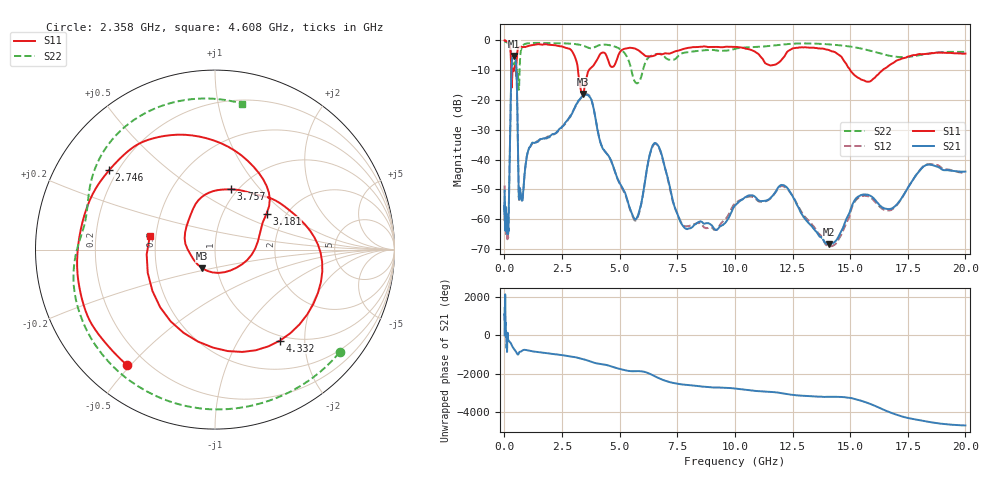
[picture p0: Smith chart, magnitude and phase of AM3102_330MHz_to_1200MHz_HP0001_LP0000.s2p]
! Date/Time: Tue, Sep 11, 2018 5:09 PM
! Network Analyzer: Agilent Technologies E8362B Rev: A.07.50.63
! Sweep from 0.010 to 20.000 GHz, 1601 Points, Sweep Type: LOG
! Power Supply: 4.950 V, 0.000 A
# Hz S DB R 50
!freq MagS11 AngS11 MagS21 AngS21 MagS12 AngS12 MagS22 AngS22
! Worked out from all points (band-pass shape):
!   1601 points, 10 MHz to 20 GHz, reference 50 ohm
!   highest |S21| = -5.20 dB at 399 MHz (marker M1); lowest = -68.4 dB at 14.07 GHz (marker M2)
!   |S21| within 3 dB of the highest: 315.2 MHz to 511 MHz (195.8 MHz wide, 47.4 % of centre)
!   lowest |S11| = -18.0 dB at 3.4 GHz (marker M3), VSWR 1.29, Z = 42.4 - j8.91 ohm
!   |S11| at or under -10 dB: 295.7 MHz to 352.7 MHz (56.97 MHz wide, 17.6 % of centre); 3.192 GHz to 3.661 GHz (469.1 MHz wide, 13.7 % of centre); 15.01 GHz to 16.4 GHz (1.393 GHz wide, 8.87 % of centre)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
!   |S22| runs from -16.6 to -0.2 dB; largest |S21 - S12| = 0.0067
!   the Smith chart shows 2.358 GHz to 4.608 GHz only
!   S11 on the Smith chart (normalised r, x): 2.358 GHz: 0.13, -0.49; 2.746 GHz: 0.17, +0.32; 3.181 GHz: 1.60, +0.73; 3.757 GHz: 0.93, +0.71; 4.332 GHz: 0.92, -1.53; 4.608 GHz: 0.46, +0.08
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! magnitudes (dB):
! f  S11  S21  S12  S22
! 10 MHz  0.0  -50.4  -48.7  -0.2
! 35.55 MHz  0.0  -58.6  -58.4  -0.3
! 126.4 MHz  -0.4  -63.2  -66.2  -0.7
! 177.1 MHz  -0.9  -63.3  -62.3  -1.1
! 399 MHz  -10.2  -5.2  -5.3  -8.1
! 447.2 MHz  -8.7  -5.7  -5.8  -7.4
! 530.6 MHz  -7.1  -11.5  -11.5  -12.5
! 635.6 MHz  -2.2  -53.3  -53.5  -15.9
! 1.59 GHz  -1.4  -33.1  -33.1  -0.8
! 2.358 GHz  -1.8  -29.9  -30.2  -0.9
! 2.746 GHz  -2.6  -26.7  -26.8  -1.0
! 3.181 GHz  -9.1  -20.6  -20.8  -1.3
! 3.4 GHz  -18.0  -18.5  -18.7  -1.7
! 3.757 GHz  -9.2  -19.6  -19.5  -2.6
! 4.332 GHz  -4.1  -36.9  -36.8  -1.4
! 4.608 GHz  -8.6  -39.9  -40.0  -1.7
! 5.652 GHz  -2.7  -60.0  -60.4  -13.7
! 6.58 GHz  -4.7  -34.5  -34.7  -4.6
! 7.845 GHz  -2.7  -63.1  -62.3  -4.0
! 12.09 GHz  -5.9  -48.5  -48.9  -1.4
! 14.07 GHz  -3.2  -68.4  -68.9  -1.3
! 20 GHz  -4.4  -44.0  -44.6  -3.8
